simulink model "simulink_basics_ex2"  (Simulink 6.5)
settings: Solver=VariableStepDiscrete  StartTime=0.0  StopTime=10  FixedStep=Tsample  RelTol=1e-3

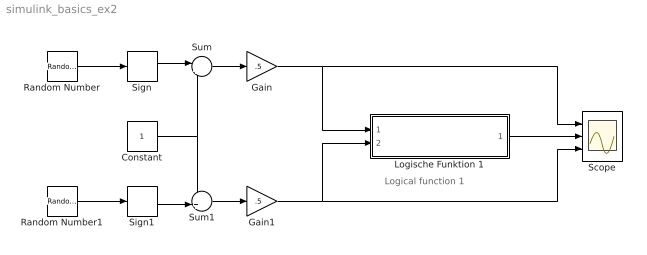
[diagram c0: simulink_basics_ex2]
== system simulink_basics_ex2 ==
  note: Logical function 1
  Constant : Constant  Value=1  OutDataType=sfix(16)  ConRadixGroup=Use specified scaling  OutScaling=2^0  SampleTime=inf  FramePeriod=inf
  Gain : Gain  Gain=.5
  Gain1 : Gain  Gain=.5
  Logische Funktion 1 : Subsystem
  Random Number : RandomNumber  SampleTime=0
  Random Number1 : RandomNumber  Seed=1  SampleTime=0
  Scope : Scope  NumInputPorts=3
  Sign : Signum
  Sign1 : Signum
  Sum : Sum  Inputs=|++
  Sum1 : Sum  Inputs=++|
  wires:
  Logische Funktion 1/1(y) -> Scope/2
  Random Number/1 -> Sign/1
  Random Number1/1 -> Sign1/1
  Gain/1 -> Logische Funktion 1/1(A), Scope/1
  Gain1/1 -> Logische Funktion 1/2(B), Scope/3
  Sign1/1 -> Sum1/2
  Sign/1 -> Sum/1
  Sum1/1 -> Gain1/1
  Constant/1 -> Sum/2, Sum1/1
  Sum/1 -> Gain/1

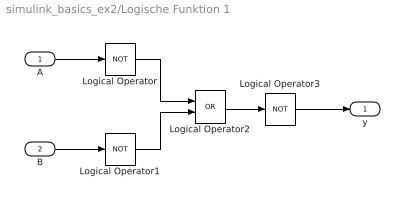
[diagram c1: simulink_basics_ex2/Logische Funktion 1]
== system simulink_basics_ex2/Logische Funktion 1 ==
  A : Inport
  B : Inport  Port=2
  Logical Operator : Logic  Operator=NOT  AllPortsSameDT=off  OutDataTypeMode=Boolean
  Logical Operator1 : Logic  Operator=NOT  AllPortsSameDT=off  OutDataTypeMode=Boolean
  Logical Operator2 : Logic  Operator=OR  AllPortsSameDT=off  OutDataTypeMode=Boolean
  Logical Operator3 : Logic  Operator=NOT  AllPortsSameDT=off  OutDataTypeMode=Boolean
  y : Outport
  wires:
  Logical Operator/1 -> Logical Operator2/1
  Logical Operator1/1 -> Logical Operator2/2
  Logical Operator2/1 -> Logical Operator3/1
  A/1 -> Logical Operator/1
  Logical Operator3/1 -> y/1
  B/1 -> Logical Operator1/1
